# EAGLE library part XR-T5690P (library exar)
T1/ISDN PRIMARY RATE FRAMER
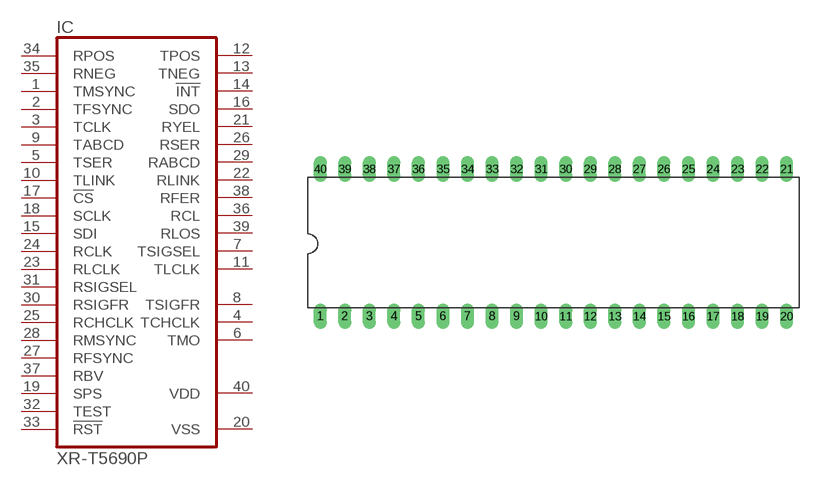
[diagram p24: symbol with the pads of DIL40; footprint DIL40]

Designator prefix IC

## XR-T5690P (OC_FARNELL: unknown; OC_NEWARK: unknown)  [DIL40]
1  TMSYNC  in
2  TFSYNC  in
3  TCLK  in
4  TCHCLK  out
5  TSER  in
6  TMO  out
7  TSIGSEL  out
8  TSIGFR  out
9  TABCD  in
10  TLINK  in
11  TLCLK  out
12  TPOS  out
13  TNEG  out
14  !INT  out
15  SDI  in
16  SDO  out
17  !CS  in
18  SCLK  in
19  SPS  in
20  VSS  pwr
21  RYEL  out
22  RLINK  out
23  RLCLK  in
24  RCLK  in
25  RCHCLK  in
26  RSER  out
27  RFSYNC  in
28  RMSYNC  in
29  RABCD  out
30  RSIGFR  in
31  RSIGSEL  in
32  TEST  in
33  !RST  in
34  RPOS  in
35  RNEG  in
36  RCL  out
37  RBV  in
38  RFER  out
39  RLOS  out
40  VDD  pwr

## Footprint DIL40 (pad centres in mm)
Dual In Line Package
drill 0.813 long: 1 -24.13,-7.62; 2 -21.59,-7.62; 3 -19.05,-7.62; 4 -16.51,-7.62; 5 -13.97,-7.62; 6 -11.43,-7.62; 7 -8.89,-7.62; 8 -6.35,-7.62; 9 -3.81,-7.62; 10 -1.27,-7.62; 11 1.27,-7.62; 12 3.81,-7.62; 13 6.35,-7.62; 14 8.89,-7.62; 15 11.43,-7.62; 16 13.97,-7.62; 17 16.51,-7.62; 18 19.05,-7.62; 19 21.59,-7.62; 20 24.13,-7.62; 21 24.13,7.62; 22 21.59,7.62; 23 19.05,7.62; 24 16.51,7.62; 25 13.97,7.62; 26 11.43,7.62; 27 8.89,7.62; 28 6.35,7.62; 29 3.81,7.62; 30 1.27,7.62; 31 -1.27,7.62; 32 -3.81,7.62; 33 -6.35,7.62; 34 -8.89,7.62; 35 -11.43,7.62; 36 -13.97,7.62; 37 -16.51,7.62; 38 -19.05,7.62; 39 -21.59,7.62; 40 -24.13,7.62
